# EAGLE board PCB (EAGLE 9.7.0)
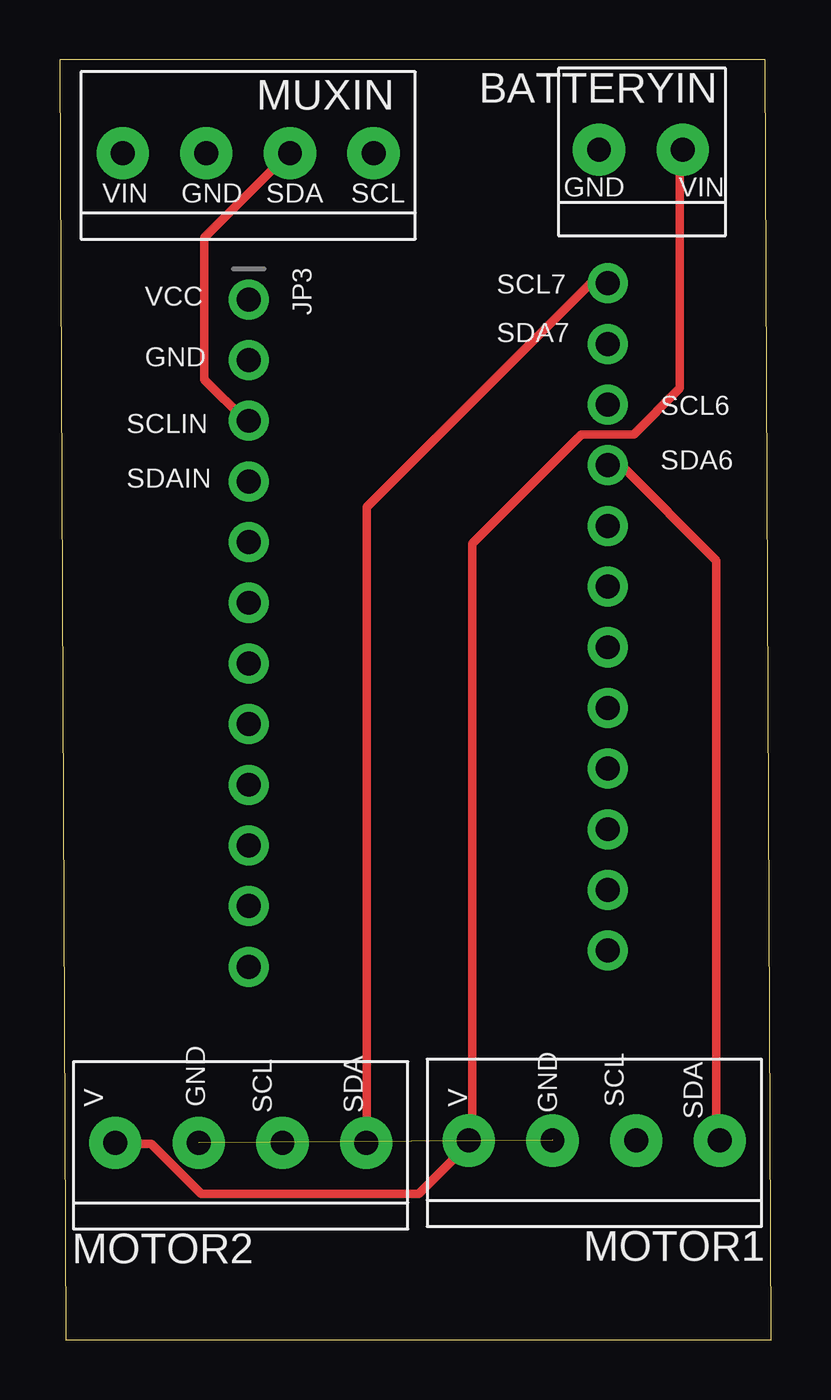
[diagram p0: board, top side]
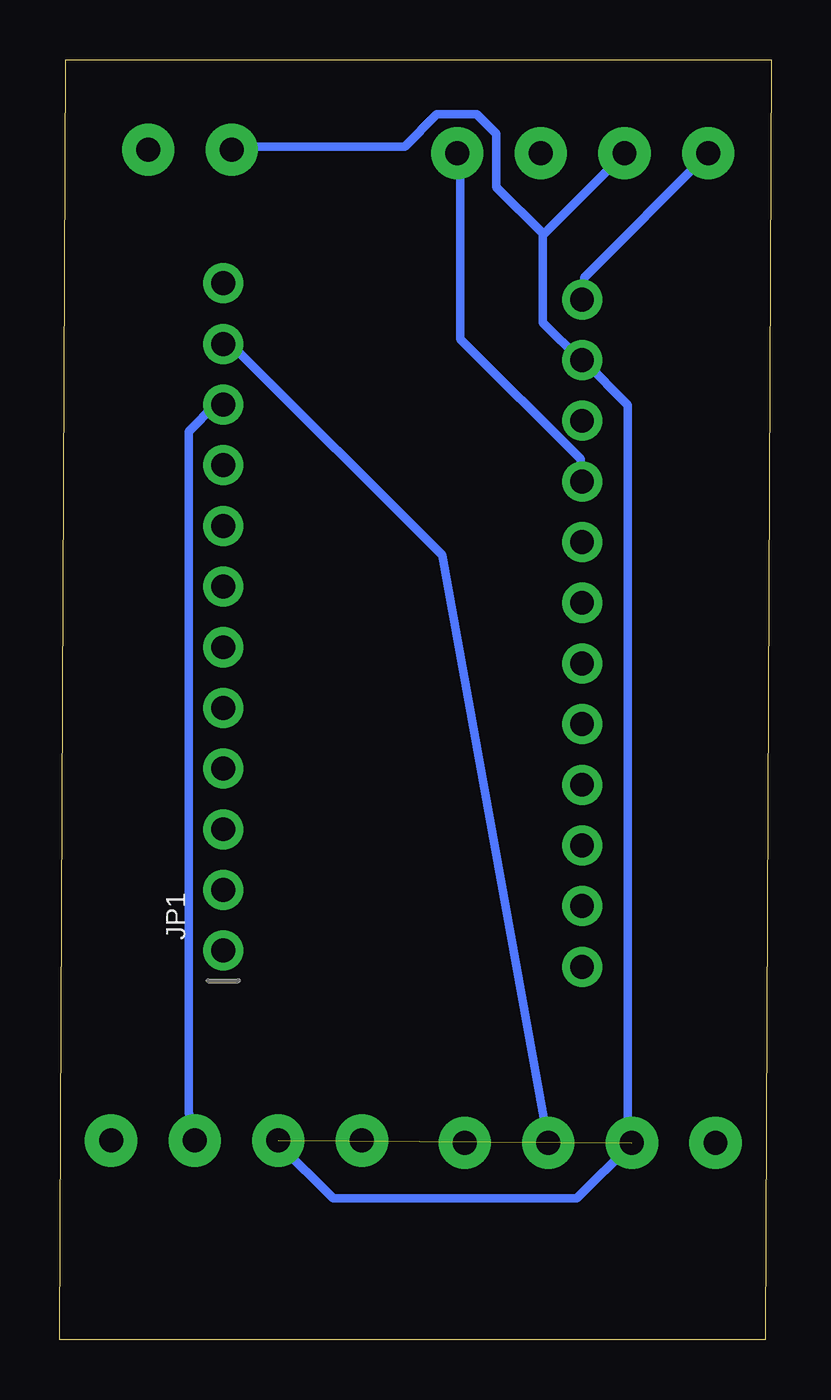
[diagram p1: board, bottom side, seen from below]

Size 29.78 x 53.6 mm. Coordinates in mm from the lower left corner, seen from the top.
Outline: 29.52,53.6 0,53.6 0.25,0 29.78,0 29.52,53.6
Copper layers (1*16): Top 0.035mm / dielectric 1.5mm / Bottom 0.035mm
Design rules "Fusion Electronics Design Rules": minimum track width 6mil, minimum drill 0.35mm, track to track 6mil, track to pad 6mil, pad to pad 6mil, via to via 6mil, smd to smd 6mil, copper to edge 40mil, drill to drill 6mil, minimum pad ring 10mil, minimum via ring 8mil, stop-mask expansion 4mil, vias tented up to drill 9999mil, thermal gap 10mil

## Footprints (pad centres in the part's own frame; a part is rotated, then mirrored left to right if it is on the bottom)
1X2-3.5MM = drill 1 pad 2.184: 1 1.8,0; 2 -1.7,0
1X12_ROUND = drill 1 pad 1.676: 1 -13.97,0; 2 -11.43,0; 3 -8.89,0; 4 -6.35,0; 5 -3.81,0; 6 -1.27,0; 7 1.27,0; 8 3.81,0; 9 6.35,0; 10 8.89,0; 11 11.43,0; 12 13.97,0
1X04-3.5MM = drill 1 pad 2.184: 1 -5.25,0; 2 -1.75,0; 3 1.75,0; 4 5.25,0

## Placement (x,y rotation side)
BATTERYIN  1X2-3.5MM  [1X2-3.5MM]  24.27,49.84 0 top
JP1  [1X12_ROUND]  22.93,30.27 90 bottom
JP3  [1X12_ROUND]  7.91,29.59 270 top
MOTOR1  1X4-3.5MM  [1X04-3.5MM]  22.38,8.34 0 top
MOTOR2  1X4-3.5MM  [1X04-3.5MM]  7.58,8.24 0 top
MUXIN  1X4-3.5MM  [1X04-3.5MM]  7.89,49.69 0 top

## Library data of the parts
BATTERYIN MOTOR1 MOTOR2 MUXIN = adafruit
JP1 JP3 = microbuilder

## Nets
0SCL: JP3.10
0SDA: JP3.9
1SCL: JP3.12
1SDA: JP3.11
2SCL: JP1.2
2SDA: JP1.1
3SCL: JP1.4
3SDA: JP1.3
4SCL: JP1.6
4SDA: JP1.5
5SCL: JP1.8
5SDA: JP1.7
6SCL: JP1.10 MOTOR1.3
6SDA: JP1.9 MOTOR1.4
7SCL: JP1.12 MOTOR2.4
7SDA: JP1.11 MOTOR2.3
A0: JP3.6
A1: JP3.7
A2: JP3.8
BAT_V: BATTERYIN.1 MOTOR1.1 MOTOR2.1
GND: BATTERYIN.2 JP3.2 MOTOR1.2 MOTOR2.2 MUXIN.2
INPUTSCL: JP3.4 MUXIN.4
INPUTSDA: JP3.3 MUXIN.3
RESET: JP3.5
VCC: JP3.1 MUXIN.1

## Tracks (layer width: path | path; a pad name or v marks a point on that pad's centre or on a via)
6SCL
  Bottom 0.356: JP1.10 23.26,39.16 24.38,38.03 24.38,9.52 MOTOR1.3
6SDA
  Top 0.356: MOTOR1.4 27.48,8.36 27.48,32.63 23.5,36.62 JP1.9
7SCL
  Top 0.356: MOTOR2.4 12.85,8.36 12.85,34.86 22.23,44.24 JP1.12
7SDA
  Bottom 0.356: MOTOR2.3 13.77,32.86 22.61,41.7 JP1.11
BAT_V
  Top 0.356: MOTOR2.1 2.34,8.21 3.83,8.21 5.92,6.12 15.03,6.12 17.12,8.21 MOTOR1.1 17.27,8.36 17.27,33.34 21.83,37.9 24.02,37.9 25.96,39.84 25.96,49.81 BATTERYIN.1
GND  (1 unrouted)
  Bottom 0.356: MOTOR1.2 20.62,8.21 18.33,5.92 8.13,5.92 5.84,8.21 6.6,8.21 6.76,8.21 5.99,8.24 5.99,39.15 7.82,40.98 JP3.2 7.97,41.02 9.55,42.6 9.55,46.26 9.52,46.28 | 9.52,46.28 9.02,46.79 8.89,46.92 6.15,49.66 MUXIN.2 | BATTERYIN.2 22.45,49.97 15.34,49.97 14,51.31 12.32,51.31 11.51,50.51 11.51,48.27 9.52,46.28
INPUTSCL
  Bottom 0.356: JP3.4 7.98,35.95 7.98,36.87 13,41.9 13,49.66 MUXIN.4
INPUTSDA
  Top 0.356: JP3.3 7.78,38.48 6.04,40.21 6.04,46.16 9.56,49.67 MUXIN.3
VCC
  Bottom 0.356: JP3.1 7.82,43.57 7.82,44.48 2.64,49.66 MUXIN.1

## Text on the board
tPlace: VIN | GND | SDA | SCL | GND | VIN | SCL7 | VCC | SDA7 | GND | SCL6 | SCLIN | SDA6 | SDAIN | V | GND | SCL | SDA | V | GND | SCL | SDA

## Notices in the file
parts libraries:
microbuilder: This work is placed in the public domain, and may be freely used for commercial and non-commercial work with the following conditions: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
